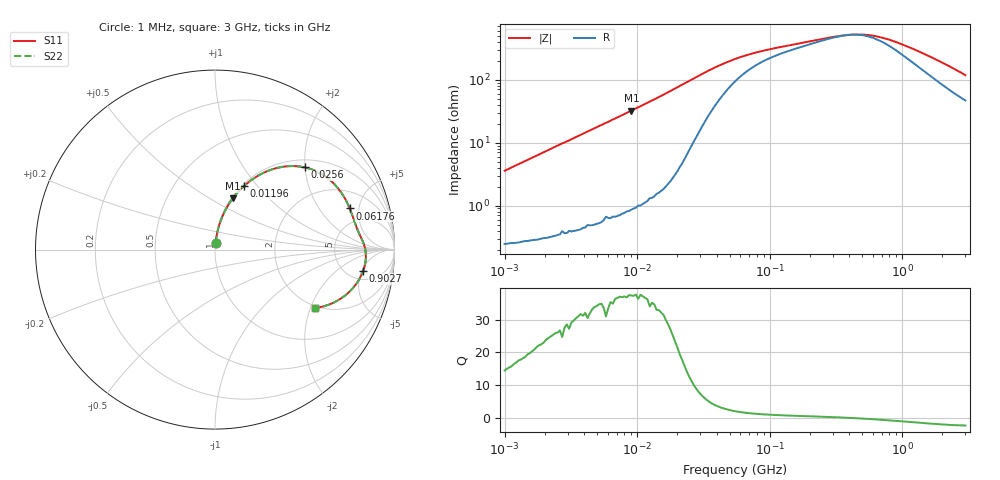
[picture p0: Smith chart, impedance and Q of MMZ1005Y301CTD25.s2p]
! S-Parameter Data Generated by TDK Corporation
! Copyright(C) 2025 TDK Corporation.
! All Rights Reserved.
! TDK P/N: MMZ1005Y301CTD25 (Chip Bead)
! Property: |Z|=300ohm at 100MHz
! Size(LxWxT): 1x0.5x0.5mm
! Model Type: s2p (Touchstone File Format Version 1.0)
! Frequency: DC=Yes Start=1MHz Stop=3000MHz 202points Log-sweep
! Model Generated on Feb. 6, 2025
! Terms and conditions regarding TDK Simulation Models:
! 1)This simulation model is being provided solely for informational
!  purposes. Please refer to the specifications of the products in
!  terms of detailed characteristics of such products.
! 2)In no event shall TDK Corporation of any of its subsidiaries be
!  liable for any loss or damage arising, directly or indirectly,
!  from any information contained in this simulation model, including,
!  but not limited to loss or damages arising from any inaccuracies,
!  omissions or errors in connection with such information.
! 3)Any and all copyrights on this simulation model are owned by
!  TDK Corporation.  Duplication or redistribution of this simulation
!  model without prior written permission from TDK Corporation
!  is prohibited.
! 4)This simulation model is subject to any modification or change
!  without any prior notice.
! 5)Neither TDK Corporation nor any of its subsidiaries shall make any
!  warranty, express or implied, including but not limited to the
!  correctness, implied warranties of merchantability and fitness for
!  a particular purpose with respect to this simulation models.
! 6)The use of this simulation model shall be deemed to have consented
!  to the terms and conditions hereof.
! Port Assignments:
!  1 ---@@@--- 2
! Applicable Conditions:
!  Temperature = 25 degC
!  DC Bias Current = 0 A
!  Small Signal Operation
# Hz S MA R 50
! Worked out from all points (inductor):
!   201 points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, 1 MHz to 3 GHz, reference 50 ohm
!   read as one part in series: L = 568 nH near 1.041 MHz
!   highest Q = 37.4 at 9.041 MHz (marker M1), where L = 565 nH
!   self-resonance near 401.5 MHz
!   S11 on the Smith chart (normalised r, x): 1 MHz: 1.00, +0.07; 11.96 MHz: 1.02, +0.86; 25.6 MHz: 1.17, +1.99; 61.76 MHz: 3.35, +4.00; 902.7 MHz: 6.81, -5.34; 3 GHz: 1.93, -2.16
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1000000  0.03562 84.0  0.9969 -2.0  0.9969 -2.0  0.03562 84.0
2055611  0.07275 83.4  0.9943 -4.2  0.9943 -4.2  0.07275 83.4
3900413  0.1364 80.3  0.9863 -7.8  0.9863 -7.8  0.1364 80.3
6058321  0.2076 76.3  0.9721 -12.0  0.9721 -12.0  0.2076 76.3
9040831  0.3036 70.8  0.9447 -17.7  0.9447 -17.7  0.3036 70.8
1.196486e7  0.3904 65.4  0.9099 -23.0  0.9099 -23.0  0.3904 65.4
1.461624e7  0.4623 60.7  0.8728 -27.5  0.8728 -27.5  0.4623 60.7
2.013356e7  0.5902 51.2  0.7803 -36.1  0.7803 -36.1  0.5902 51.2
2.559965e7  0.6775 42.6  0.6789 -42.4  0.6789 -42.4  0.6775 42.6
3.670325e7  0.7546 29.8  0.51 -47.4  0.51 -47.4  0.7546 29.8
5.477226e7  0.7815 19.3  0.3681 -44.5  0.3681 -44.5  0.7815 19.3
6.176144e7  0.785 17.0  0.3384 -42.6  0.3384 -42.6  0.785 17.0
1.039275e8  0.7955 10.1  0.2574 -32.7  0.2574 -32.7  0.7955 10.1
2.136344e8  0.817 4.6  0.1969 -19.5  0.1969 -19.5  0.817 4.6
3.453811e8  0.8336 1.2  0.1675 -6.0  0.1675 -6.0  0.8336 1.2
4.570858e8  0.8399 -1.1  0.1611 5.8  0.1611 5.8  0.8399 -1.1
6.049187e8  0.8419 -3.7  0.1691 18.9  0.1691 18.9  0.8419 -3.7
8.005644e8  0.838 -6.8  0.1948 30.5  0.1948 30.5  0.838 -6.8
9.0272e8  0.8341 -8.2  0.2114 34.4  0.2114 34.4  0.8341 -8.2
1.243477e9  0.8153 -12.7  0.2719 41.2  0.2719 41.2  0.8153 -12.7
1.782824e9  0.7734 -18.9  0.3666 43.0  0.3666 43.0  0.7734 -18.9
3e9  0.6464 -30.2  0.5486 36.4  0.5486 36.4  0.6464 -30.2
